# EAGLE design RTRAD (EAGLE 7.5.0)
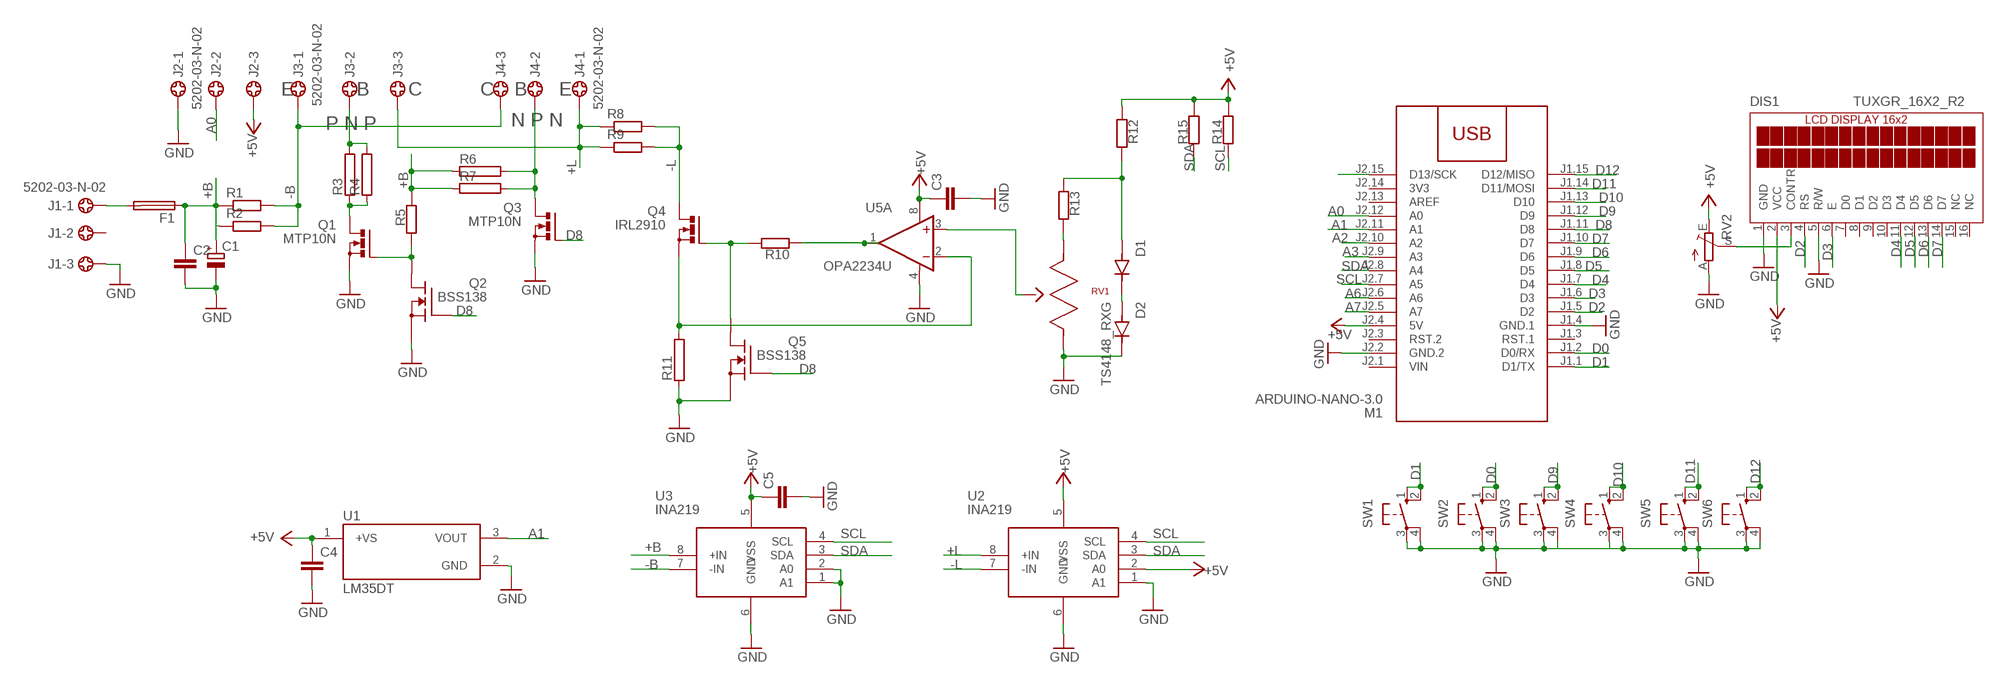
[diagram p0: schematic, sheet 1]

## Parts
C1  CPOL-EUSMCD  [SMC_D]
C2  C-EUC1206  [C1206]
C3  C-EUC1206  [C1206]
C4  C-EUC1206  [C1206]
C5  C-EUC1206  [C1206]
D1  TS4148_RXG  [DIO_TS4148_RXG]
D2  TS4148_RXG  [DIO_TS4148_RXG]
DIS1  TUXGR_16X2_R2  [TUXGR_16X2_R2]
F1  SH22,5A  [SH22,5A]
J1  5202-03-N-02  [5202-03-N-02]
J2  5202-03-N-02  [5202-03-N-02]
J3  5202-03-N-02  [5202-03-N-02]
J4  5202-03-N-02  [5202-03-N-02]
M1  ARDUINO-NANO-3.0  [ARDUINO-NANO-3.0]
Q1  MTP10N  BUZ11BV  [TO220BV]
Q2  BSS138  [SOT23]
Q3  MTP10N  BUZ11BV  [TO220BV]
Q4  IRL2910  BUZ11BV  [TO220BV]
Q5  BSS138  [SOT23]
R1  R-EU_R2512W  [R2512W]
R2  R-EU_R2512W  [R2512W]
R3  RKH216-8  [KH216-8]
R4  RKH216-8  [KH216-8]
R5  R-EU_R1206  [R1206]
R6  RKH216-8  [KH216-8]
R7  RKH216-8  [KH216-8]
R8  R-EU_R2512W  [R2512W]
R9  R-EU_R2512W  [R2512W]
R10  R-EU_R1206  [R1206]
R11  RKH216-8  [KH216-8]
R12  R-EU_R1206  [R1206]
R13  R-EU_R1206  [R1206]
R14  R-EU_R1206  [R1206]
R15  R-EU_R1206  [R1206]
RV1  PTV09A-4025F-A103  [PTV09]
RV2  TRIM_EU-B64W  [B64W]
SW1  10-XX  [B3F-10XX]
SW2  10-XX  [B3F-10XX]
SW3  10-XX  [B3F-10XX]
SW4  10-XX  [B3F-10XX]
SW5  10-XX  [B3F-10XX]
SW6  10-XX  [B3F-10XX]
U1  LM35DT  [TO254P1016X457X1955-3]
U2  INA219  [SO08]
U3  INA219  [SO08]
U5  OPA2234U  [SO08]

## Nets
+5V: C3.1 C4.1 C5.1 DIS1.2(VCC) J2.3 M1.J2.4(5V) R12.2 R14.1 R15.1 RV2.E U1.1(+VS) U2.2(A0) U2.5(VSS) U3.5(VSS) U5.8(A:V+)
+B: C1.+ C2.1 F1.1 R1.1 R2.1 R5.1 R6.1 R7.1 U3.8(+IN)
+L: J3.3 J4.1 R8.1 R9.1 U2.8(+IN)
-B: J3.1 J4.3 R1.2 R2.2 U3.7(-IN)
-L: Q4.D R8.2 R9.2 U2.7(-IN)
A0: J2.2 M1.J2.12(A0)
A1: M1.J2.11(A1) U1.3(VOUT)
A2: M1.J2.10(A2)
A3: M1.J2.9(A3)
A6: M1.J2.6(A6)
A7: M1.J2.5(A7)
D0: M1.J1.2(D0/RX) SW2.1(S) SW2.2(S1)
D1: M1.J1.1(D1/TX) SW1.1(S) SW1.2(S1)
D2: DIS1.4(RS) M1.J1.5(D2)
D3: DIS1.6(E) M1.J1.6(D3)
D4: DIS1.11(D4) M1.J1.7(D4)
D5: DIS1.12(D5) M1.J1.8(D5)
D6: DIS1.13(D6) M1.J1.9(D6)
D7: DIS1.14(D7) M1.J1.10(D7)
D8: M1.J1.11(D8) Q2.3(G) Q3.G Q5.3(G)
D9: M1.J1.12(D9) SW3.1(S) SW3.2(S1)
D10: M1.J1.13(D10) SW4.1(S) SW4.2(S1)
D11: M1.J1.14(D11/MOSI) SW5.1(S) SW5.2(S1)
D12: M1.J1.15(D12/MISO) SW6.1(S) SW6.2(S1)
D13: M1.J2.15(D13/SCK)
GND: C1.- C2.2 C3.2 C4.2 C5.2 D2.C(K) DIS1.1(GND) DIS1.5(R/W) J1.3 J2.1 M1.J1.4(GND.1) M1.J2.2(GND.2) Q1.S Q2.1(S) Q3.S Q5.1(S) R11.1 RV1.3 RV2.A SW1.3(P) SW1.4(P1) SW2.3(P) SW2.4(P1) SW3.3(P) SW3.4(P1) SW4.3(P) SW4.4(P1) SW5.3(P) SW5.4(P1) SW6.3(P) SW6.4(P1) U1.2(GND) U2.1(A1) U2.6(GND) U3.1(A1) U3.2(A0) U3.6(GND) U5.4(A:V-)
N$1: J3.2 R3.2 R4.2
N$2: Q1.G Q2.2(D) R5.2
N$3: Q1.D R3.1 R4.1
N$4: F1.2 J1.1
N$5: J4.2 Q3.D R6.2 R7.2
N$7: Q4.S R11.2 U5.2(A:-IN)
N$8: Q4.G Q5.2(D) R10.1
N$9: R10.2 U5.1(A:OUT)
N$10: RV1.2 U5.3(A:+IN)
N$11: R13.1 RV1.1
N$12: D1.C(K) D2.A
N$13: D1.A R12.1 R13.2
N$14: DIS1.3(CONTR) RV2.S
SCL: M1.J2.7(A5) R14.2 U2.4(SCL) U3.4(SCL)
SDA: M1.J2.8(A4) R15.2 U2.3(SDA) U3.3(SDA)
Unconnected: DIS1.7(D0) DIS1.8(D1) DIS1.9(D2) DIS1.10(D3) DIS1.15(NC) DIS1.16(NC) J1.2 M1.J1.3(RST.1) M1.J2.3(RST.2) M1.J2.13(AREF) U5.5(B:+IN) U5.6(B:-IN) U5.7(B:OUT)

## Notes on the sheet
- E | B | C | C | B | E
- P N P | N P N

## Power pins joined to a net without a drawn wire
3V3: M1.J2.14(3V3)
VIN: M1.J2.1(VIN)

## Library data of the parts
C1 = rcl:CPOL-EU: POLARIZED CAPACITOR, European symbol
C2-C5 = rcl:C-EU: CAPACITOR, European symbol
D1 D2 = TS4148_RXG:TS4148_RXG: Check availability Check availability Check availability; AVAILABILITY: In Stock; CHECK_PRICES: https://www.snapeda.com/parts/TS4148%20RXG/Taiwan+Semiconductor/view-part/?ref=eda; DESCRIPTION: 1206 (Ceramics) 75V 0.15A Switching Diode & Array; MF: Taiwan Semiconductor; MP: TS4148 RXG; PACKAGE: 1206-2 Taiwan Semiconductor; PRICE: None; SNAPEDA_LINK: https://www.snapeda.com/parts/TS4148%20RXG/Taiwan+Semiconductor/view-part/?ref=snap
DIS1 = display-lcd:TUXGR_16X2_R2: Tuxgraphics LCD display 16x2 characters reflective, without background light Source: tuxgr_12x2_r2.pdf; OC_FARNELL: unknown; OC_NEWARK: unknown
F1 = fuse:SH22,5A: FUSE HOLDER; MPN: 0031.7701.11; OC_FARNELL: unknown; OC_NEWARK: 04F1224
J1-J4 = con-ebyelectro:5202-03-N-02: Barrier Blocks Sreies 5202 Source: http://www.ebyelectro.com/PDF/5202-XX-N-02.pdf; OC_FARNELL: unknown; OC_NEWARK: unknown
M1 = diy-modules:ARDUINO-NANO-3.0: Arduino Nano 3.0 and compatible devices More details available here: https://www.arduino.cc/en/Main/ArduinoBoardNano Click here to find device on ebay.com
Q1 Q3 Q4 = transistor-power:BUZ11: N-CHANNEL MOS FET
Q2 Q5 = transistor-fet:BSS138
R1 R2 R5 R8-R10 R12-R15 = rcl:R-EU_: RESISTOR, European symbol
R3 R4 R6 R7 R11 = resistor-power:R: Power Resitor; OC_FARNELL: unknown; OC_NEWARK: unknown
RV1 = PTV09A-4025F-A103:PTV09A-4025F-A103: 10k Ohm 1 Gang Logarithmic Through Hole, Snap In Potentiometer None 1 Turn Carbon 0.05W, 1/20W PC Pins, Board Locks Check availability; AVAILABILITY: In Stock; CHECK_PRICES: https://www.snapeda.com/parts/PTV09A-4025F-A103/Bourns/view-part/?ref=eda; DESCRIPTION: 10k Ohm 1 Gang Logarithmic Through Hole, Snap In Potentiometer None 1.0 Kierros Carbon 0.05W, 1/20W PC Pins, Board Locks; MF: Bourns; MP: PTV09A-4025F-A103; PACKAGE: None; PRICE: None; PURCHASE-URL: https://www.snapeda.com/api/url_track_click_mouser/?unipart_id=1440680&manufacturer=Bourns&part_name=PTV09A-4025F-A103&search_term=ptv09a; SNAPEDA_LINK: https://www.snapeda.com/parts/PTV09A-4025F-A103/Bourns/view-part/?ref=snap
RV2 = pot:TRIM_EU-: POTENTIOMETER
SW1-SW6 = switch-omron:10-XX: OMRON SWITCH; MPN: B3F-1000; OC_FARNELL: 176432; OC_NEWARK: 36M3542
U1 = LM35DT-H:LM35DT: Check availability; AVAILABILITY: In Stock; CHECK_PRICES: https://www.snapeda.com/parts/LM35DT/Texas+Instruments/view-part/?ref=eda; DESCRIPTION: ±0.5°C 4V-30V, Temperature sensor with analog output 3-TO-220 0 to 100; MF: Texas Instruments; MP: LM35DT; PACKAGE: TO-220-3 Texas Instruments; PRICE: None; SNAPEDA_LINK: https://www.snapeda.com/parts/LM35DT/Texas+Instruments/view-part/?ref=snap
U2 U3 = burr-brown:INA219: Bidirectional Current/Power Monitor With I2C Interface
U5 = burr-brown:OPA2234: Operational Amplifier; MF: TEXAS INSTRUMENTS; MPN: OPA2234U; OC_FARNELL: 1212441; OC_NEWARK: 96K4523

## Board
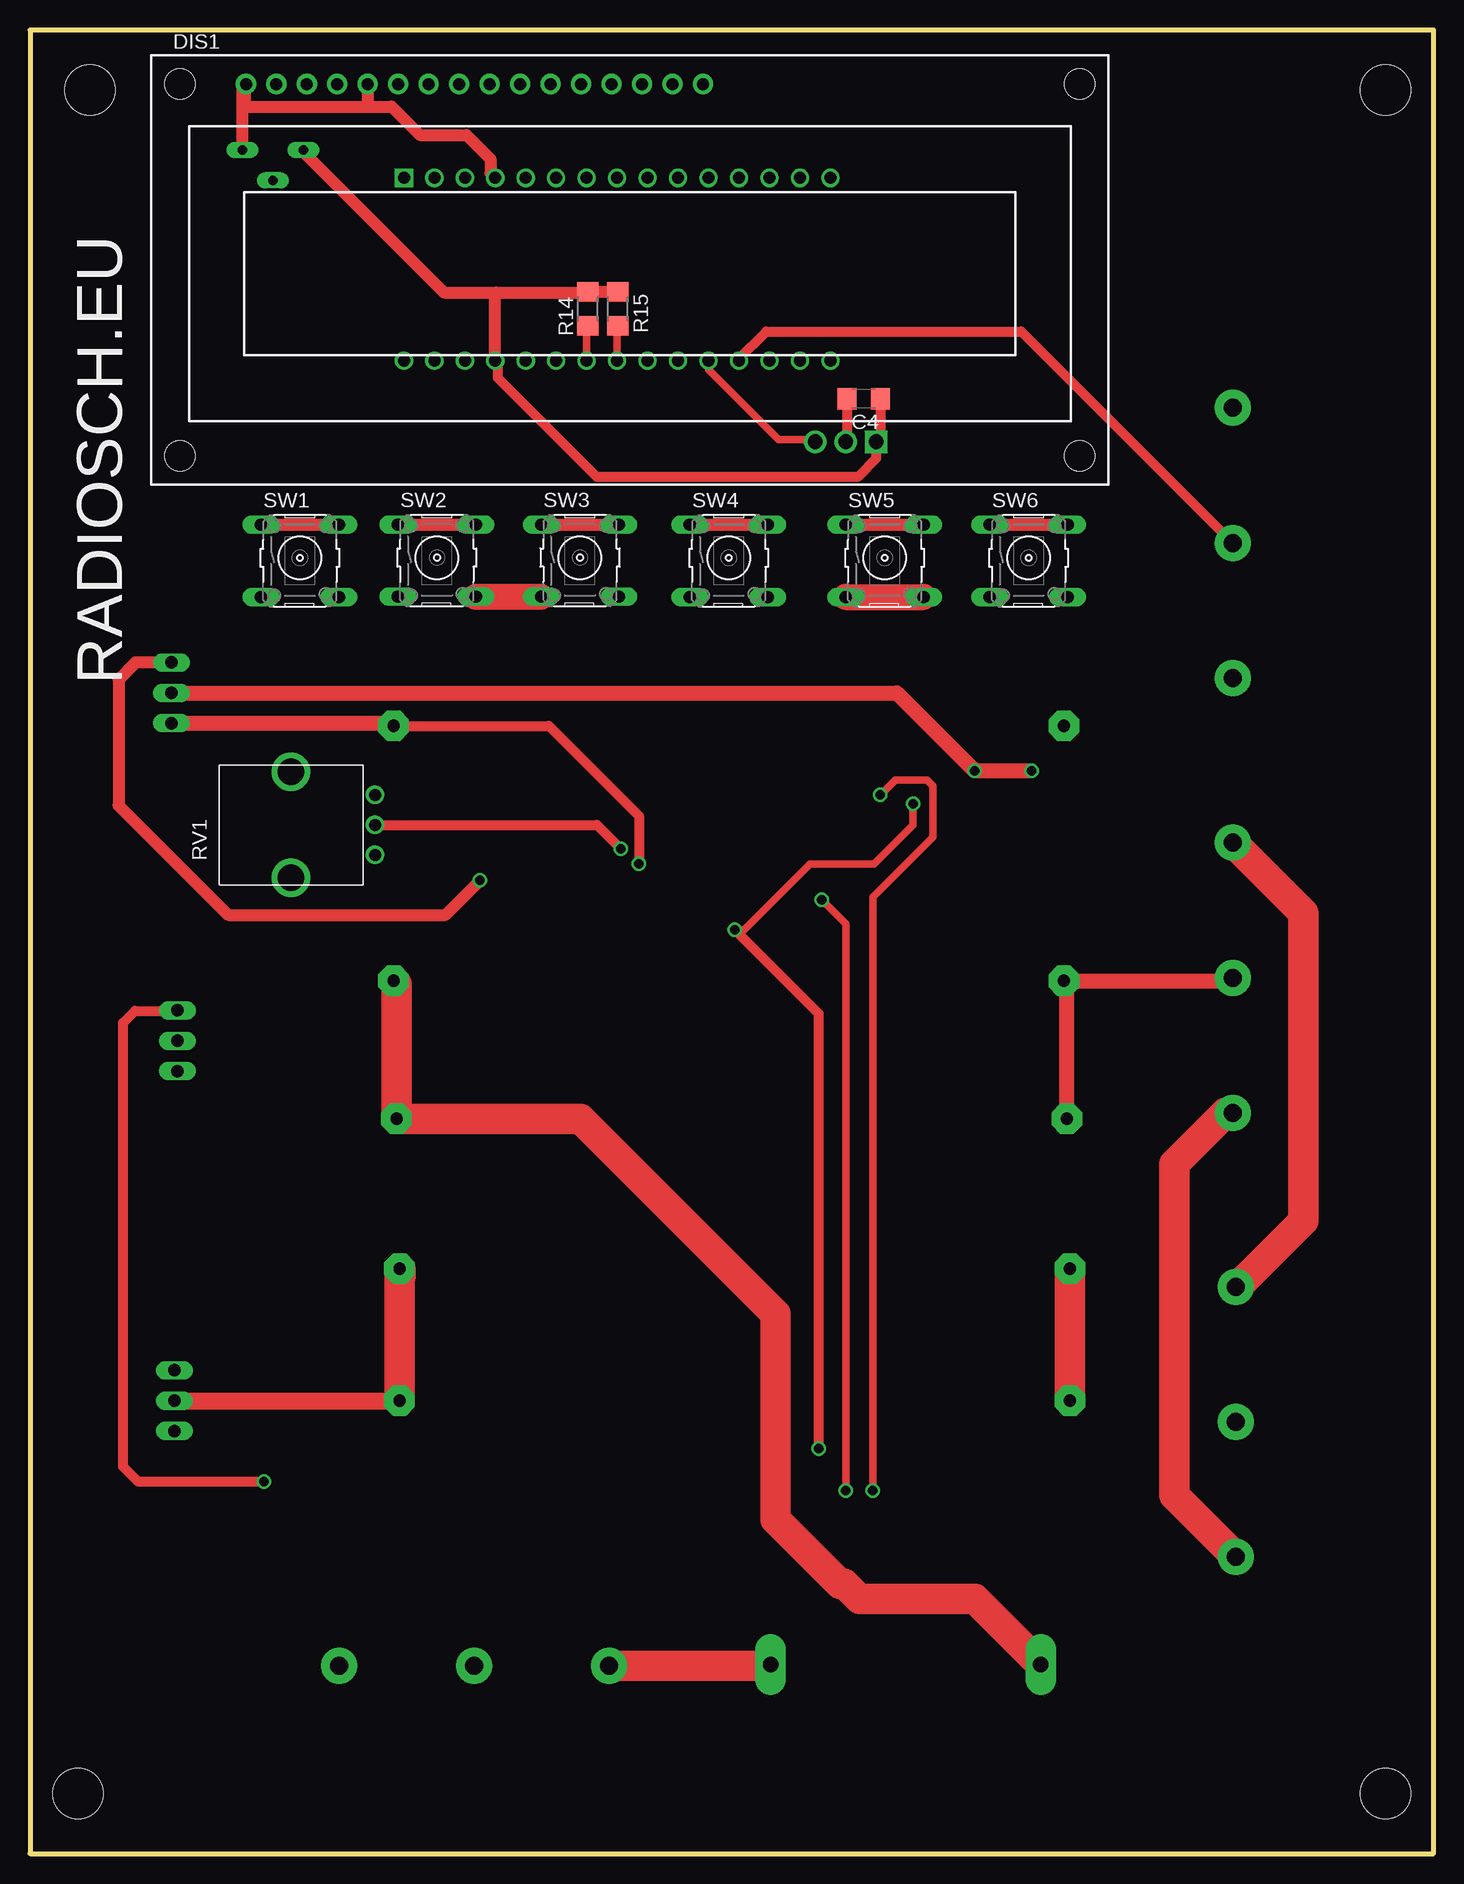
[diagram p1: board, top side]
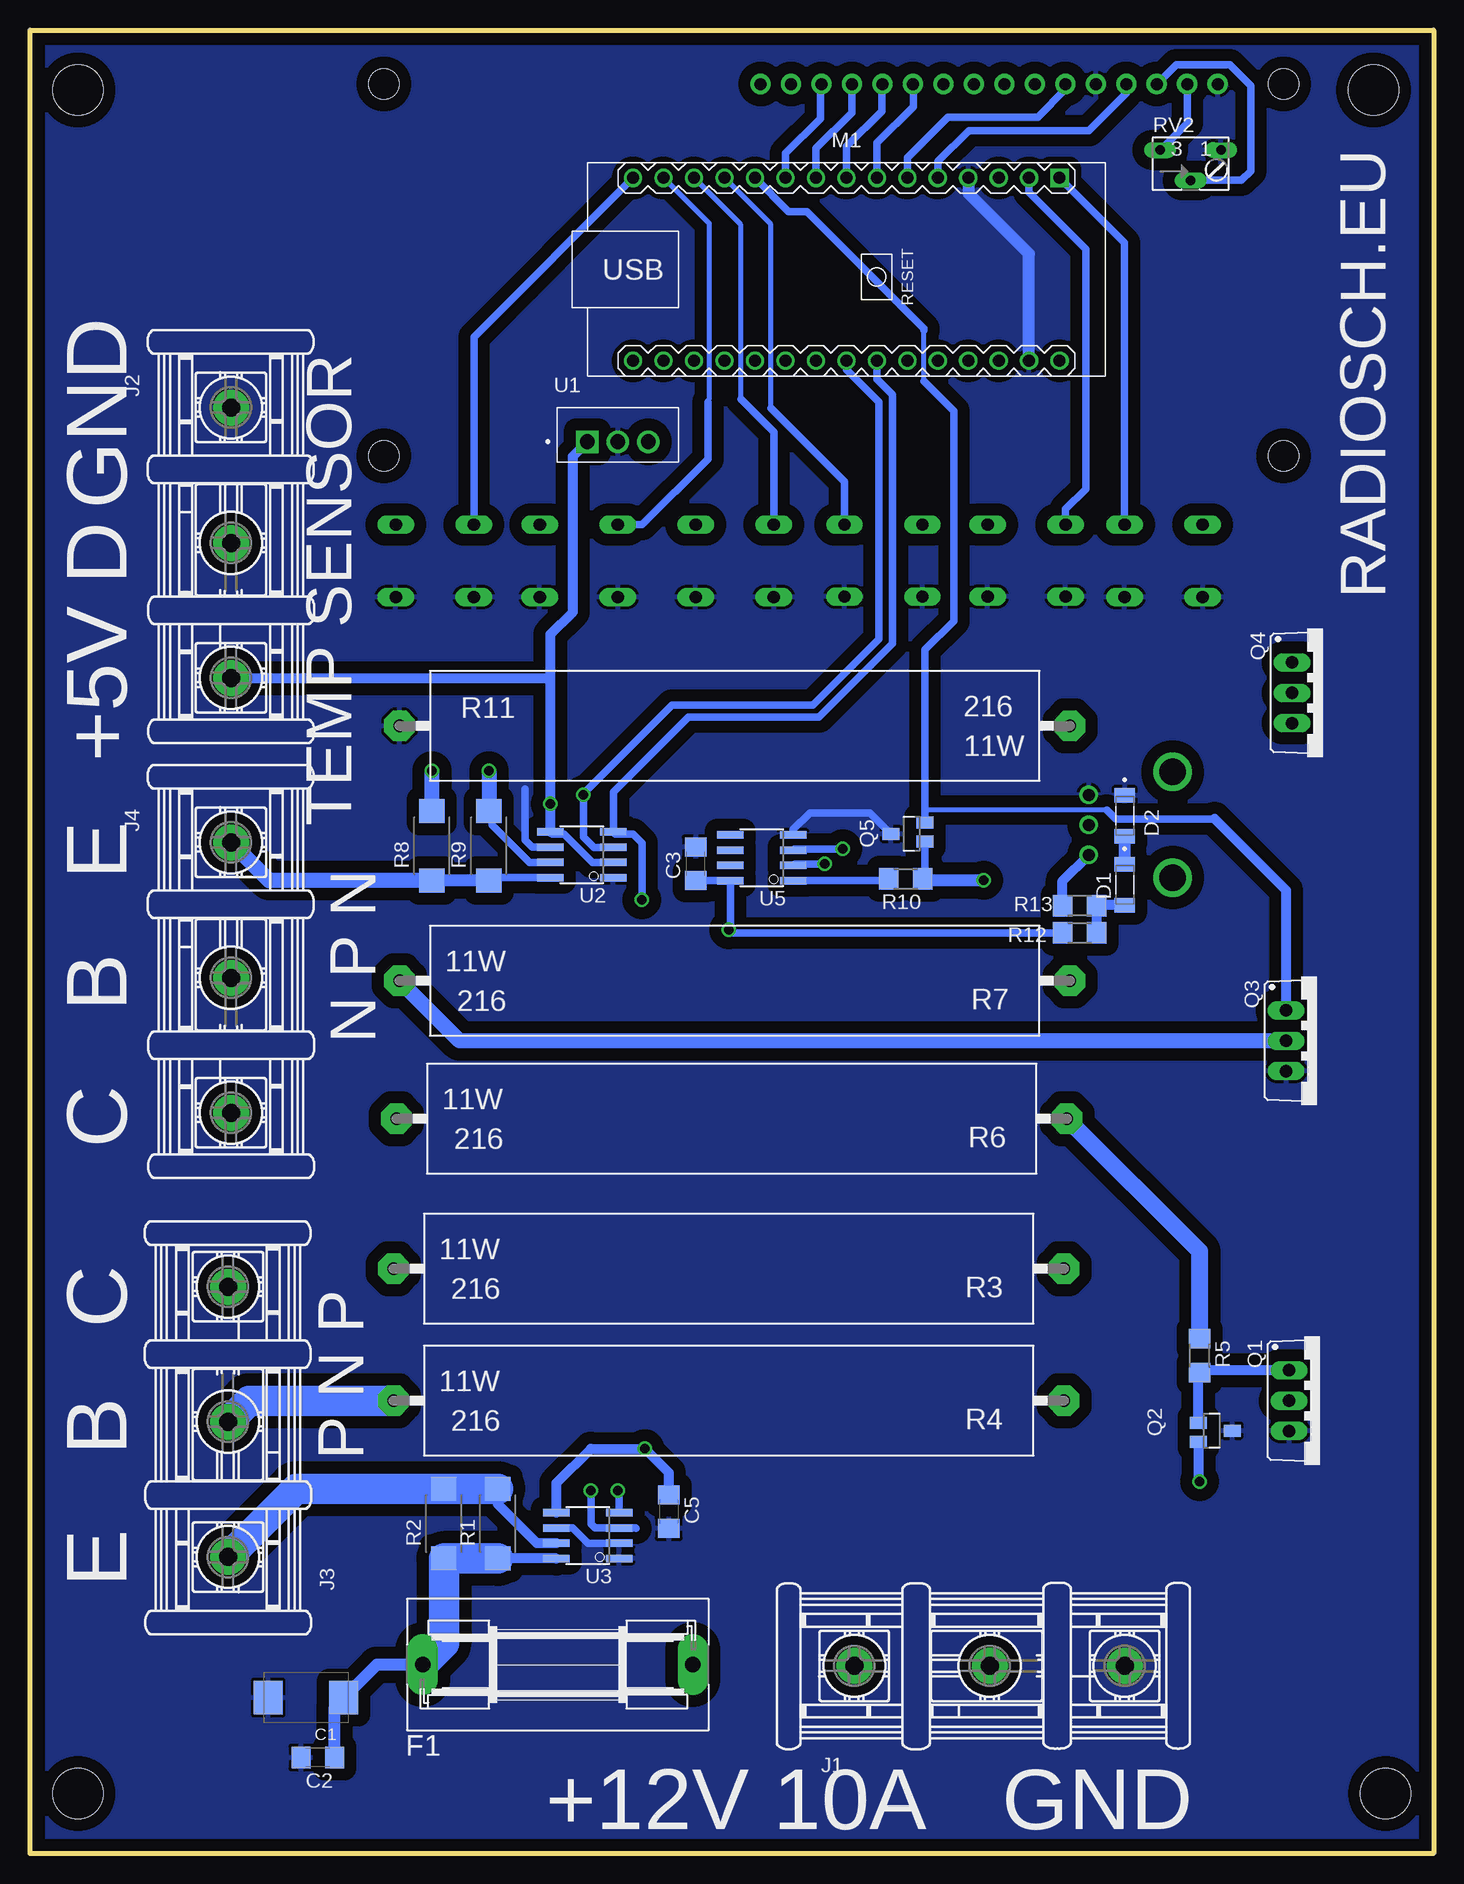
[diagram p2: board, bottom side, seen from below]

Size 117 x 152 mm. Coordinates in mm from the lower left corner, seen from the top.
Outline: 0,0 117,0 117,152 0,152 0,0
Copper layers (1*16): Top 0.035mm / dielectric 1.5mm / Bottom 0.035mm
Design rules "default": minimum track width 10mil, minimum drill 24mil, track to track 8mil, track to pad 8mil, pad to pad 8mil, via to via 8mil, smd to smd 8mil, copper to edge 40mil, drill to drill 8mil, minimum pad ring 10mil, minimum via ring 8mil, stop-mask expansion 4mil, vias tented up to drill 0mil, thermal gap 10mil
Holes 4.2 mm at 5,147 4,5 113,147 113,5

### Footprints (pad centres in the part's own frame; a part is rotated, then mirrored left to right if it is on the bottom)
SMC_D = smd 2.4 x 2.8: + -3.15,0; - 3.15,0
C1206 = smd 1.6 x 1.8: 1 -1.4,0; 2 1.4,0
DIO_TS4148_RXG = smd 1.2 x 1.7: A 1.7,0; C -1.7,0
TUXGR_16X2_R2 = drill 1 pad 1.676: 1 -32,15.5; 2 -29.46,15.5; 3 -26.92,15.5; 4 -24.38,15.5; 5 -21.84,15.5; 6 -19.3,15.5; 7 -16.76,15.5; 8 -14.22,15.5; 9 -11.68,15.5; 10 -9.14,15.5; 11 -6.6,15.5; 12 -4.06,15.5; 13 -1.52,15.5; 14 1.02,15.5; 15 3.56,15.5; 16 6.1,15.5 | hole 2.5: -37.5,-15.5; 37.5,-15.5; -37.5,15.5; 37.5,15.5
SH22,5A = drill 1.321 pad 2.54 long: 1 -11.252,0; 2 11.252,0
5202-03-N-02 = drill 1.5 pad 3: 1 -9.29,0; 2 2,0; 3 13.25,0
ARDUINO-NANO-3.0 = drill 1 square: J1.1 17.78,7.62 | drill 1: J1.2 15.24,7.62; J1.3 12.7,7.62; J1.4 10.16,7.62; J1.5 7.62,7.62; J1.6 5.08,7.62; J1.7 2.54,7.62; J1.8 0,7.62; J1.9 -2.54,7.62; J1.10 -5.08,7.62; J1.11 -7.62,7.62; J1.12 -10.16,7.62; J1.13 -12.7,7.62; J1.14 -15.24,7.62; J1.15 -17.78,7.62; J2.1 17.78,-7.62; J2.2 15.24,-7.62; J2.3 12.7,-7.62; J2.4 10.16,-7.62; J2.5 7.62,-7.62; J2.6 5.08,-7.62; J2.7 2.54,-7.62; J2.8 0,-7.62; J2.9 -2.54,-7.62; J2.10 -5.08,-7.62; J2.11 -7.62,-7.62; J2.12 -10.16,-7.62; J2.13 -12.7,-7.62; J2.14 -15.24,-7.62; J2.15 -17.78,-7.62
TO220BV = drill 1.016 long: D 0,-2.54; G -2.54,-2.54; S 2.54,-2.54
SOT23 = smd 1 x 1.4: 1 0,1.735; 2 -0.632,-1.1; 3 0.95,-1.1
R2512W = smd 2 x 2.1: 1 -2.896,0; 2 2.896,0
KH216-8 = drill 1.016 pad 2.54 octagon: 1 -27.94,0; 2 27.94,0
R1206 = smd 1.6 x 1.803: 1 -1.422,0; 2 1.422,0
PTV09 = drill 1: 1 -2.5,0; 2 0,0; 3 2.5,0 | drill 2.2: NC1 -4.4,7; NC2 4.4,7
B64W = drill 0.813 long: A 2.54,0; E -2.54,0; S 0,-2.54
B3F-10XX = drill 1.016 long: 1 -3.251,2.761; 2 3.251,2.761; 3 -3.251,-3.261; 4 3.251,-3.261
TO254P1016X457X1955-3 = drill 1.24 square: 1 -2.54,-0.573 | drill 1.24: 2 0,-0.573; 3 2.54,-0.573
SO08 = smd 0.61 x 2.21: 1 -1.905,-2.616; 2 -0.635,-2.616; 3 0.635,-2.616; 4 1.905,-2.616; 5 1.905,2.616; 6 0.635,2.616; 7 -0.635,2.616; 8 -1.905,2.616

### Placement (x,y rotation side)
C1  94,13 180 bottom
C2  93,8 180 bottom
C3  61.5,82.5 90 bottom
C4  69.5,121.25 180 top
C5  63.75,28.5 270 bottom
D1  25.75,80.75 270 bottom
D2  25.75,86.5 270 bottom
DIS1  50,132 0 top
F1  73,15.75 0 bottom
J1  39,15.64 0 bottom
J2  100.25,111.25 270 bottom
J3  100.5,34 90 bottom
J4  100.25,75 270 bottom
M1  48.95,132.05 0 bottom
Q1  9.5,37.75 270 bottom
Q2  18.5,35.25 270 bottom
Q3  9.75,67.75 270 bottom
Q4  9.25,96.75 270 bottom
Q5  43.5,85 90 bottom
R1  78,27.5 90 bottom
R2  82.5,27.5 90 bottom
R3  58.75,48.75 180 bottom
R4  58.75,37.75 180 bottom
R5  19.5,41.5 270 bottom
R6  58.5,61.25 180 bottom
R7  58.25,72.75 180 bottom
R8  83.5,84 90 bottom
R9  78.75,84 90 bottom
R10  44,81.25 180 bottom
R11  58.25,94 0 bottom
R12  29.5,76.75 180 bottom
R13  29.5,79 0 bottom
R14  46.5,128.75 270 top
R15  49,128.75 270 top
RV1  28.75,85.75 90 top
RV2  20.25,142 0 bottom
SW1  22.5,108 0 top
SW2  33.92,108.02 0 top
SW3  45.85,108.02 0 top
SW4  58.25,108 0 top
SW5  71.25,108 0 top
SW6  83.25,108 0 top
U1  68,118.25 0 bottom
U2  71,83.25 90 bottom
U3  70.5,26.5 90 bottom
U5  56,83 90 bottom

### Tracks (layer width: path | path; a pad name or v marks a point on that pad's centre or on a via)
+5V  (via drill 0.8)
  Top 0.61: v58.75,77 59.5,77 65,82.5 70.37,82.5 73.62,85.75 v73.62,87.5
  Top 0.813: M1.J2.4 39,124.22 39,123 47.25,114.75 69,114.75 70.54,116.29 U1.1 70.9,118.04 C4.1 | v65.75,33.75 65.75,70 v58.75,77
  Top 1.016: RV2.E 22.79,141.83 34.5,130.12 38.88,130.12 | 38.88,130.12 46.45,130.12 R14.1 R15.1 | M1.J2.4 38.79,130.04 38.88,130.12
  Bottom 0.61: DIS1.2 20.54,144.25 RV2.E | U2.2 70.11,82.62 72.5,85 73.46,85 U2.5 | R12.2 58.5,76.75 v58.75,77 58.62,77.13 U5.8 C3.1
  Bottom 0.813: U2.5 v73.62,87.5 73.62,98 | 73.62,98 73.62,101.63 71.75,103.5 71.75,116.47 U1.1 | J2.3 73.62,98 | U3.5 73.12,30.88 70.25,33.75 v65.75,33.75 63.75,31.75 C5.1
+B
  Top 2.54: F1.1 78.75,21.25 69.12,21.25 67.88,22.5 67.5,22.5 62.12,27.88 62.12,45 45.88,61.25 R6.1 30.56,72.5 R7.1
  Bottom 0.813: U3.8 R1.1
  Bottom 1.016: F1.1 88.1,15.75 C1.+ 91.6,12.25 C2.1
  Bottom 1.422: R5.1 19.5,50.19 R6.1
  Bottom 2.54: R1.1 R2.1 82.5,17.5 F1.1
+L
  Top 2.54: J3.3 100.62,47.25 106.12,52.75 106.12,78.41 J4.1
  Bottom 0.61: U2.8 78.51,81.34 R9.1
  Bottom 1.016: R9.1 R8.1
  Bottom 1.27: R8.1 97.06,81.1 J4.1
-B
  Top 2.54: J4.3 99.62,61.75 95.38,57.5 95.38,29.84 J3.1
  Bottom 0.813: U3.7 74.74,25.86 78,29.12 R1.2
  Bottom 2.54: J3.1 94.81,30.4 R2.2 R1.2
-L  (via drill 0.8)
  Top 1.27: Q4.D 72.25,96.75 v78.75,90.25 v83.5,90.25
  Bottom 0.61: U2.7 75.36,82.62 78.5,85.75 78.5,86.65 R9.2
  Bottom 1.27: v78.75,90.25 R9.2 | R8.2 v83.5,90.25
A0
  Top 0.813: M1.J2.12 59.11,124.61 61.38,126.88 82.62,126.88 J2.2
A1
  Top 0.61: M1.J2.11 56.57,123.68 62.38,117.88 65.26,117.88 U1.3
D0
  Top 1.016: SW2.1 SW2.2
  Bottom 0.61: SW2.1 30.67,112.08 29,113.75 29,133.75 33.75,138.5 33.75,139.63 M1.J1.2
D1
  Top 1.016: SW1.1 SW1.2
  Bottom 0.61: SW1.2 25.75,134.25 M1.J1.1
D2
  Bottom 0.61: M1.J1.5 41.33,141.05 38.75,143.62 28.75,143.62 25.62,146.75 DIS1.4
D3
  Bottom 0.61: DIS1.6 30.7,147.05 33,144.75 40.5,144.75 43.88,141.38 M1.J1.6
D4
  Bottom 0.61: M1.J1.7 46.41,142.59 43.38,145.62 43.38,147.47 DIS1.11
D5
  Bottom 0.61: M1.J1.8 48.95,142.3 46,145.25 46,147.44 DIS1.12
D6
  Bottom 0.61: M1.J1.9 51.49,142.13 48.5,145.12 48.5,147.48 DIS1.13
D7
  Bottom 0.61: M1.J1.10 54.03,141.72 51.12,144.62 51.12,147.39 DIS1.14
D8  (via drill 0.8)
  Top 0.813: v19.5,31 9,31 7.75,32.25 7.75,69.25 8.75,70.25 12.25,70.25 Q3.G
  Bottom 0.406: 42.5,122.75 42.5,127 | 27.25,87 42.27,87
  Bottom 0.61: Q5.3 42.4,87.12 | 42.4,87.12 42.4,100.35 40,102.75 40,120.25 42.5,122.75 | 42.5,127 42.5,127.12 52.25,136.88 53.77,136.88 M1.J1.11 | 18.25,86.25 26.5,86.25 27.25,87 | 42.27,87 42.4,87.12
  Bottom 0.813: Q3.G 12.29,80.29 18.25,86.25 | Q2.3 19.6,31.1 v19.5,31
D9
  Top 1.016: SW3.1 SW3.2
  Bottom 0.406: 55.25,120.5 55.25,135.81 M1.J1.12
  Bottom 0.61: SW3.2 49.1,114.35 55.25,120.5
D10
  Top 1.016: SW4.1 SW4.2
  Bottom 0.406: 57.75,121.25 57.75,135.77 M1.J1.13
  Bottom 0.61: SW4.1 55,118.5 57.75,121.25
D11
  Top 1.016: SW5.1 SW5.2
  Bottom 0.406: 60.5,121 60.5,121.12 60.38,121.25 60.38,135.86 M1.J1.14
  Bottom 0.61: SW5.1 65.99,110.76 60.5,116.25 60.5,121
D12
  Top 1.016: SW6.1 SW6.2
  Bottom 0.61: SW6.1 80,126.4 M1.J1.15
GND
  Top 0.813: C4.2 68.1,117.78 U1.2
  Top 1.016: M1.J1.4 38.38,140.08 38.38,141.25 36.38,143.25 32.5,143.25 30.12,145.62 28.38,145.62 | RV2.A 17.71,147.21 DIS1.1 18,147.38 17.88,147.25 17.88,145.62 28.38,145.62 | DIS1.5 28.16,145.84 28.38,145.62
  Top 2.184: SW2.4 SW3.3 | SW5.3 SW5.4
  Bottom 0.61: U5.4 53.38,85.37 52,86.75 46.98,86.75 Q5.1 | U2.6 75.14,83.88 75.75,84.5 75.75,88.75 | U3.6 71.76,27.14 70.5,25.88 67.89,25.88 U3.2
  Bottom 1.016: M1.J2.2 33.71,133.33 38.75,138.38 38.75,139.63 M1.J1.4
  pour Bottom (isolate 1.016): 1,152 116,151 116.25,-0.25 1.25,0.75
N$1
  Top 2.54: R3.2 R4.2
  Bottom 2.54: R4.2 98.75,37.75 J3.2
N$2
  Bottom 0.813: Q1.G 19.29,40.29 R5.2 19.6,39.98 Q2.2
N$3
  Top 1.422: Q1.D R4.1
  Top 2.54: R4.1 30.81,48.06 30.88,48.12 30.88,48.69 R3.1
N$4
  Top 2.54: J1.1 61.64,15.64 F1.2
N$5
  Top 1.27: R6.2 86.44,72.44 86.75,72.75 | 86.75,72.75 R7.2 | 86.75,72.75 100,72.75 J4.2
  Bottom 1.27: Q3.D 81.19,67.75 R7.2
N$7  (via drill 0.8)
  Top 0.813: R11.2 43.25,94 50.75,86.5 v50.75,82.5
  Top 1.27: Q4.S 30.1,94.21 R11.2
  Bottom 0.61: v50.75,82.5 53.25,82.5 U5.2
N$8  (via drill 0.8)
  Top 1.016: Q4.G 8.79,99.29 7.38,97.88 7.38,87.38 16.5,78.25 34.62,78.25 v37.5,81.12
  Bottom 0.61: Q5.2 42.4,81.43 R10.1
  Bottom 1.016: v37.5,81.12 42.45,81.12 R10.1
N$9
  Bottom 0.61: U5.1 45.58,81.09 R10.2
N$10  (via drill 0.8)
  Top 0.813: RV1.2 47.25,85.75 v49.25,83.75
  Bottom 0.61: v49.25,83.75 53.27,83.75 U5.3
N$11
  Bottom 0.813: R13.1 30.92,81.08 RV1.1
N$12
  Bottom 1.016: D1.C D2.A
N$13
  Bottom 0.813: D1.A 28.03,79.05 R13.2 R12.1
N$14
  Bottom 0.61: RV2.S 16.04,139.46 15.25,140.25 15.25,147.38 17,149.12 21.45,149.12 DIS1.3
SCL  (via drill 0.8)
  Top 0.61: M1.J2.7 46.41,127.24 R14.2 | v68,30.25 68,77.5 v66,79.5
  Bottom 0.61: M1.J2.7 46.41,122.91 45.12,121.62 45.12,100.88 51.25,94.75 62.12,94.75 68.38,88.5 U2.4 68.23,85 66.75,85 66,84.25 v66,79.5 | U3.4 67.88,30.13 v68,30.25
SDA  (via drill 0.8)
  Top 0.61: M1.J2.8 48.95,127.28 R15.2 | v70.25,30.25 70.25,79.75 75.25,84.75 75.25,89 74.75,89.5 72.12,89.5 v70.88,88.25
  Bottom 0.61: M1.J2.8 48.95,123.7 46.25,121 46.25,101.25 51.75,95.75 63.5,95.75 69.38,89.88 70.88,88.38 v70.88,88.25 70.88,84.75 70,83.88 68.39,83.88 U2.3 | 66.5,27.12 66.51,27.14 U3.3 69.89,27.14 70.25,27.5 v70.25,30.25

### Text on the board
tPlace: RADIOSCH.EU
bPlace: GND | TEMP SENSOR | D | RADIOSCH.EU | +5V | E | N P N | B | C | C | P N P | B | E | GND | +12V 10A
